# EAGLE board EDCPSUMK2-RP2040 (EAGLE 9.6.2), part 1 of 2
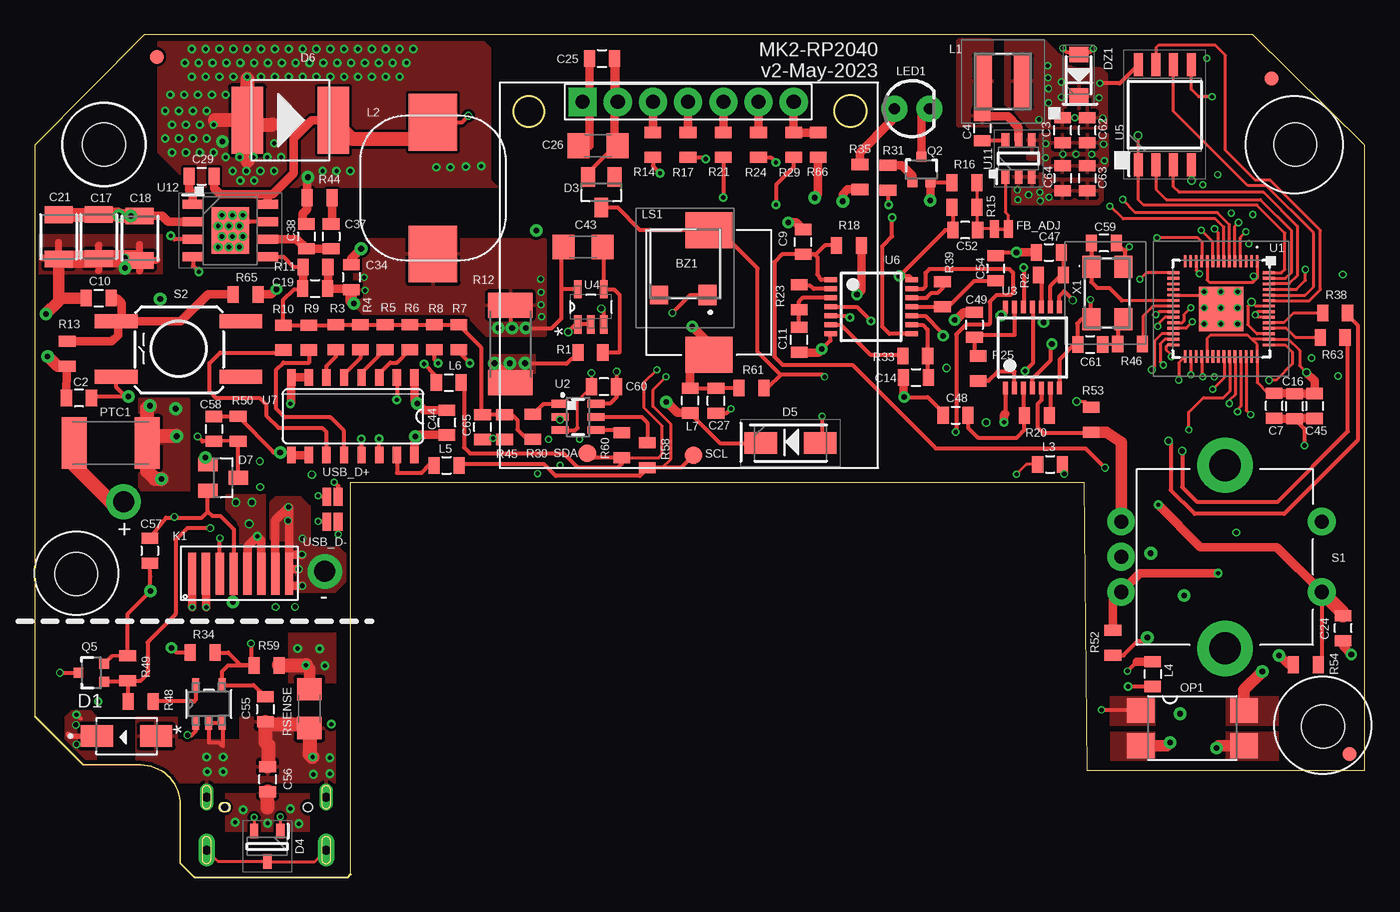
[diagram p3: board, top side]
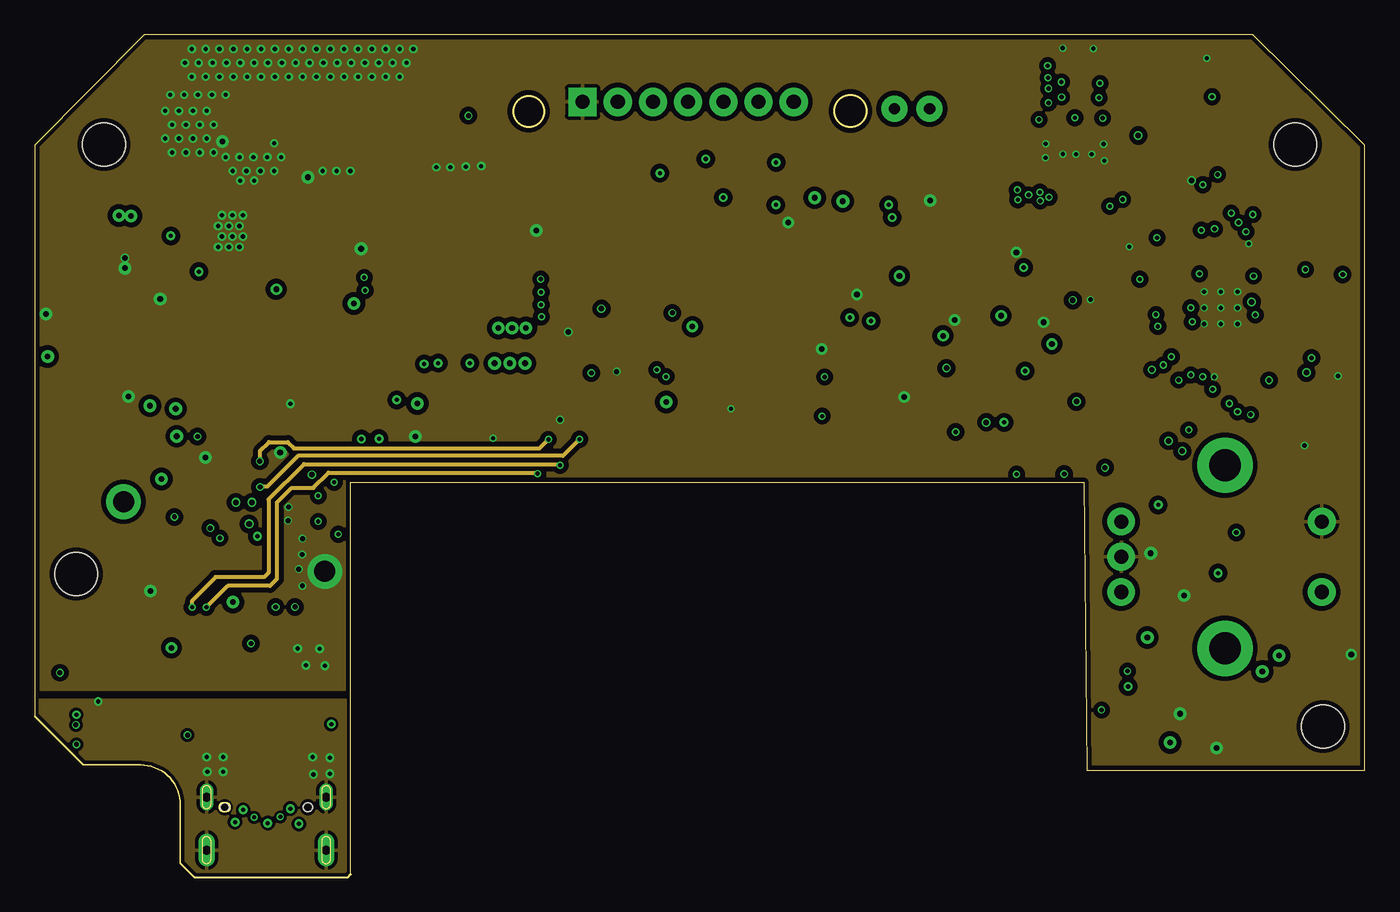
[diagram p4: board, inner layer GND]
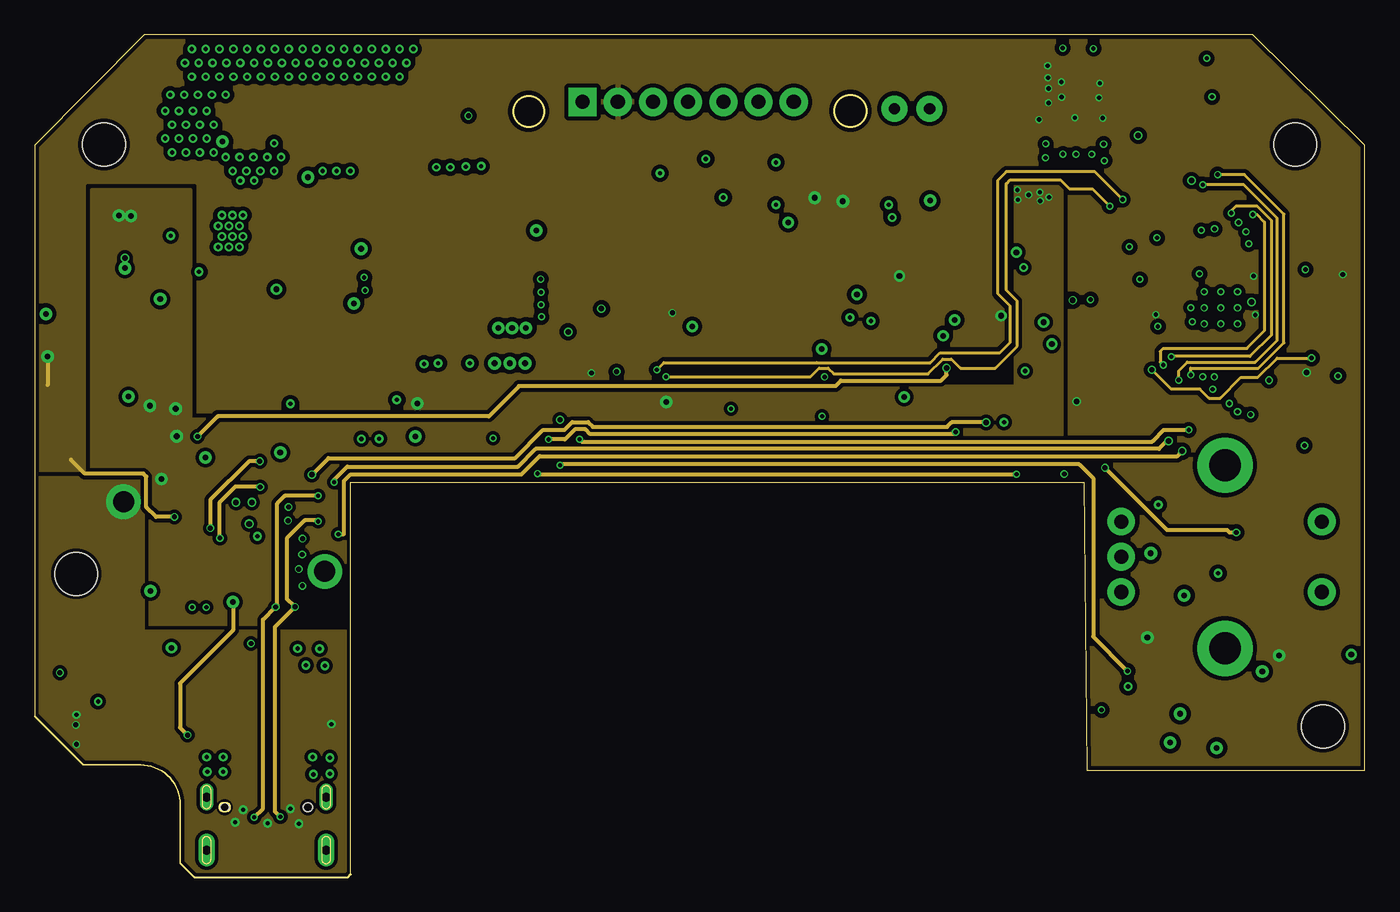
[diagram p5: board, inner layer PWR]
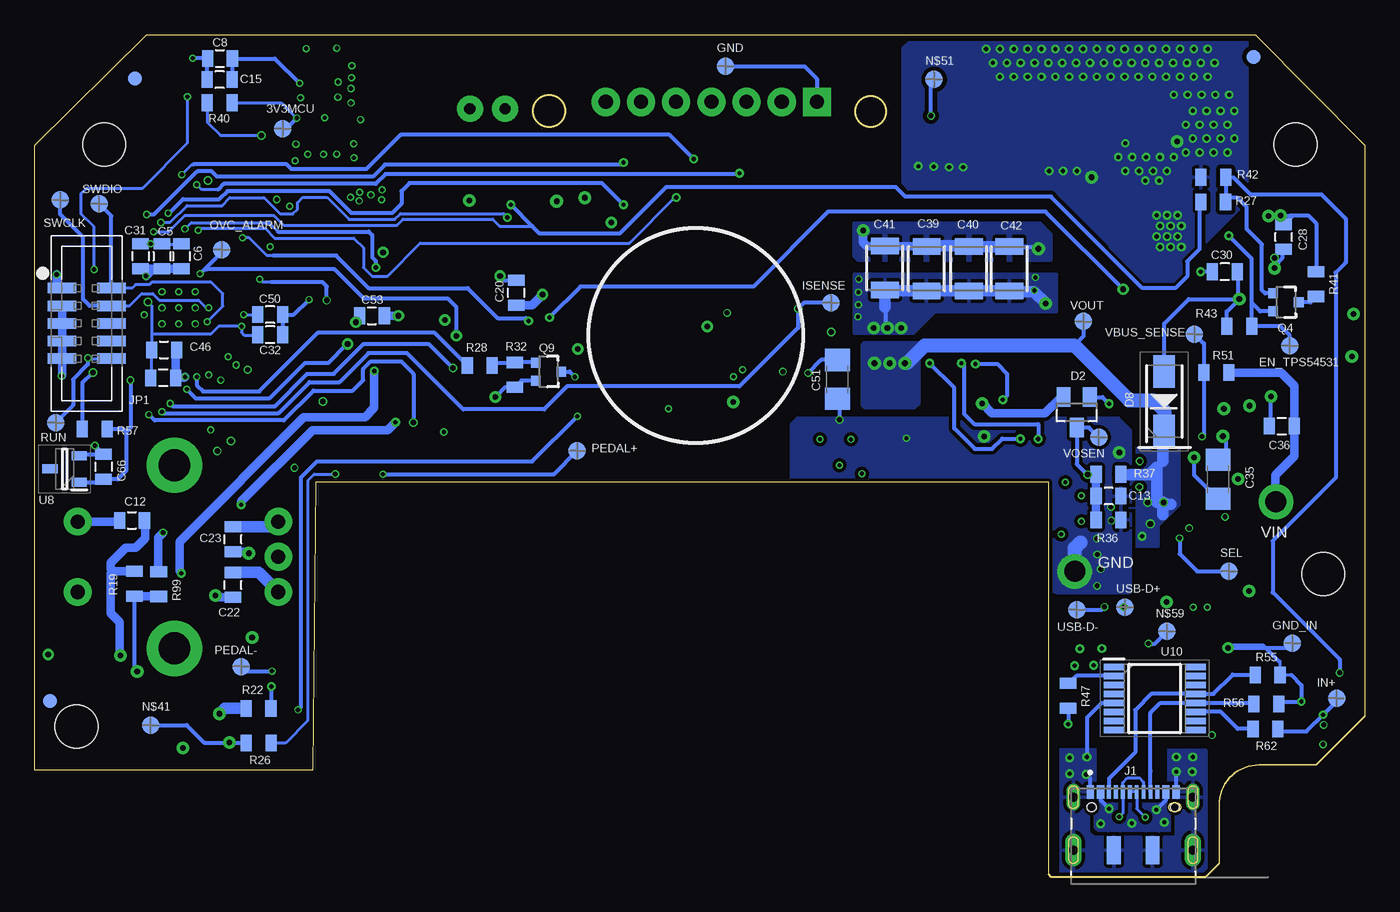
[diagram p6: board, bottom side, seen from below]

Size 96 x 60.8 mm. Coordinates in mm from the lower left corner, seen from the top.
Outline: 96,7.7 96,52.8 87.9,60.8 7.9,60.8 0,52.8 0,11.6 3.5,8.1 7.62,8.1 arc-90 10.5,5.22 10.5,1 11.5,0 22.6,0 22.8,0.2 22.8,28.5 75.71,28.5 75.92,7.7 96,7.7
Outline: circle at 35.64,55.26 radius 1.09
Outline: circle at 58.87,55.29 radius 1.14
Copper layers (1*2*15*16): Top 0.035mm / dielectric 0.2mm / GND 0.0175mm / dielectric 0.3mm / PWR 0.0175mm / dielectric 0.2mm / Bottom 0.035mm
Design rules "SeeedStudio_4layer_DRU_no_angle_20140221 *": minimum track width 8mil, minimum drill 12mil, track to track 8mil, track to pad 8mil, pad to pad 8mil, via to via 8mil, smd to smd 0mil, copper to edge 10mil, drill to drill 8mil, minimum pad ring 6mil, minimum via ring 4mil, stop-mask expansion 4mil, vias tented up to drill 25mil, thermal gap 10mil
Net classes: 1 vcc: width 0.254 mm
Holes 3.1 mm at 4.98,52.88 90.98,52.88 2.98,21.88 92.98,10.88
tRestrict: area 0.4,19.3 to 5.4,24.3; area 2.5,50.4 to 7.5,55.4; area 88.5,50.4 to 93.5,55.4; area 90.5,8.4 to 95.5,13.4
bRestrict: area 90.5,8.4 to 95.5,13.4; area 88.5,50.4 to 93.5,55.4; area 2.5,50.4 to 7.5,55.4; area 0.4,19.4 to 5.4,24.4

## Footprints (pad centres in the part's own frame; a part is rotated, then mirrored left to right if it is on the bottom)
TESTPAD_B1,27 = smd 1.27 x 1.27: TP 0,0
PKMCS0909 = smd 2.6 x 3.4: 1 -4.5,0; 2 4.5,0
0805 = smd 0.8 x 1.2: 1 -0.9,0; 2 0.9,0
1210 = smd 1.2 x 2: 1 -1.6,0; 2 1.6,0
1206 = smd 1.6 x 1.8: 1 -1.4,0; 2 1.4,0
DIOM4325X244N = smd 2.33 x 1.55: A 2.135,0; C -2.135,0
SOT23 = smd 1 x 1.4: 1 -0.95,-1.1; 2 0.95,-1.1; 3 0,1.1
SOT95P230X110-3N = smd 1.05 x 0.6: 1 -1.1,0.95; 2 -1.1,-0.95; 3 1.1,0
DIOM5226X244N = smd 2.35 x 1.55: 1 -2.15,0; 2 2.15,0
DO-214AB = smd 2.286 x 4.8: 1 -3.1,0; 2 3.1,0
SODFL3518X115N = smd 1.12 x 1.37: 1 -1.5,0; 2 1.5,0
SMT-JUMPER_2_NC_TRACE_NO-SILK = smd 0.635 x 1.27: 1 -0.508,0; 2 0.508,0
FIDUCIAL-1X2 = smd 1 x 1: 1 0,0
JAE_DX07S016JA1R1500 = smd 0.52 x 1: 1 -3.1,1.1; 2 -2.35,1.1; 11 2.35,1.1; 12 3.1,1.1 | smd 0.27 x 1: 3 -1.75,1.1; 4 -1.25,1.1; 5 -0.75,1.1; 6 -0.25,1.1; 7 0.25,1.1; 8 0.75,1.1; 9 1.25,1.1; 10 1.75,1.1 | smd 1 x 2: S1 -1.4,-3.1; S2 1.4,-3.1 | drill 0.65 long: S3 -4.32,0.725; S4 4.32,0.725 | drill 0.65 pad 1.2 long: S5 -4.32,-3.1; S6 4.32,-3.1 | hole 0.6: 3,0 | hole 0.63: 3,0; -3,0
OLED_LCD = drill 1.016 pad 2.032 square: 1 -7.42,13.7 | drill 1.016 pad 2.032: 2 -4.88,13.7; 3 -2.34,13.7; 4 0.2,13.7; 5 2.74,13.7; 6 5.28,13.7; 7 7.82,13.7
20021521-00010T1LF = smd 0.76 x 2.05: 1 -2.54,-1.78; 2 -2.54,1.78; 3 -1.27,-1.78; 4 -1.27,1.78; 5 0,-1.78; 6 0,1.78; 7 1.27,-1.78; 8 1.27,1.78; 9 2.54,-1.78; 10 2.54,1.78
FLEX8 = smd 0.6 x 3: 1 0.8,2.05; 2 1.8,2.05; 3 2.8,2.05; 4 3.8,2.05; 5 4.8,2.05; 7 5.8,2.05; 8 6.8,2.05; 9 7.8,2.05
NRS4018T100MDGJ = smd 1.2 x 3.7: 1 -1.4,0; 2 1.4,0
WE-LHMI = smd 4.1 x 3.5: 1 -4.75,0; 2 4.75,0
LED3MM = drill 0.813 pad 1.88: A -1.27,0; K 1.27,0
SMT0540SR = smd 1.5 x 1.3: 1 -2.25,-1.6; 2 2.25,-1.6 | smd 1.3 x 1.3: 3 -2.25,1.9
SMD4 = smd 1.78 x 2: 1 -1.27,-3.725; 2 1.27,-3.725; 3 1.27,3.725; 4 -1.27,3.725
1812L = smd 1.8 x 3.7: 1 -2.6,0; 2 2.65,0
SOT323 = smd 0.7 x 0.7: 1 -0.65,-0.925; 2 0.65,-0.925; 3 0,0.925
R2512 = smd 1.8 x 3.2: 1 -2.8,0; 2 2.8,0
ROTARY_ENC_PLAIN = drill 1.016 pad 2: A 7.493,-2.54; B 7.493,2.54; C 7.493,0; SW+ -6.985,2.54; SW- -6.985,-2.54 | drill 2.286 pad 4: P$3 0,6.604; P$4 0,-6.604
TAC_SW_SMD_KSC931G = smd 3.1 x 1: 1 -4.5,2; 2 4.5,2; 3 -4.5,-2; 4 4.5,-2
RP2040TR7 = smd 0.875 x 0.2: 1 -3.438,2.6; 2 -3.438,2.2; 3 -3.438,1.8; 4 -3.438,1.4; 5 -3.438,1; 6 -3.438,0.6; 7 -3.438,0.2; 8 -3.438,-0.2; 9 -3.438,-0.6; 10 -3.438,-1; 11 -3.438,-1.4; 12 -3.438,-1.8; 13 -3.438,-2.2; 14 -3.438,-2.6; 29 3.438,-2.6; 30 3.438,-2.2; 31 3.438,-1.8; 32 3.438,-1.4; 33 3.438,-1; 34 3.438,-0.6; 35 3.438,-0.2; 36 3.438,0.2; 37 3.438,0.6; 38 3.438,1; 39 3.438,1.4; 40 3.438,1.8; 41 3.438,2.2; 42 3.438,2.6 | smd 0.2 x 0.875: 15 -2.6,-3.438; 16 -2.2,-3.438; 17 -1.8,-3.438; 18 -1.4,-3.438; 19 -1,-3.438; 20 -0.6,-3.438; 21 -0.2,-3.438; 22 0.2,-3.438; 23 0.6,-3.438; 24 1,-3.438; 25 1.4,-3.438; 26 1.8,-3.438; 27 2.2,-3.438; 28 2.6,-3.438; 43 2.6,3.438; 44 2.2,3.438; 45 1.8,3.438; 46 1.4,3.438; 47 1,3.438; 48 0.6,3.438; 49 0.2,3.438; 50 -0.2,3.438; 51 -0.6,3.438; 52 -1,3.438; 53 -1.4,3.438; 54 -1.8,3.438; 55 -2.2,3.438; 56 -2.6,3.438 | smd 3.2 x 3.2: 57 0,0
SOT23-6 = smd 0.55 x 1.2: 1 0.95,1.3; 2 0,1.3; 3 -0.95,1.3; 4 -0.95,-1.3; 5 0,-1.3; 6 0.95,-1.3
TSSOP14 = smd 0.35 x 0.9: 1 -1.95,-2.925; 2 -1.3,-2.925; 3 -0.65,-2.925; 4 0,-2.925; 5 0.65,-2.925; 6 1.3,-2.925; 7 1.95,-2.925; 8 1.95,2.925; 9 1.3,2.925; 10 0.65,2.925; 11 0,2.925; 12 -0.65,2.925; 13 -1.3,2.925; 14 -1.95,2.925
SOT95P280X145-5N = smd 1.321 x 0.559: 1 -1.27,0.94; 2 -1.27,0; 3 -1.27,-0.94; 4 1.27,-0.94; 5 1.27,0.94
SOIC127P790X216-8N = smd 1.65 x 0.65: 1 -3.6,1.905; 2 -3.6,0.635; 3 -3.6,-0.635; 4 -3.6,-1.905; 5 3.6,-1.905; 6 3.6,-0.635; 7 3.6,0.635; 8 3.6,1.905
SO16 = smd 0.6 x 1.2: 1 -4.445,-2.8; 2 -3.175,-2.8; 3 -1.905,-2.8; 4 -0.635,-2.8; 5 0.635,-2.8; 6 1.905,-2.8; 7 3.175,-2.8; 8 4.445,-2.8; 9 4.445,2.8; 10 3.175,2.8; 11 1.905,2.8; 12 0.635,2.8; 13 -0.635,2.8; 14 -1.905,2.8; 15 -3.175,2.8; 16 -4.445,2.8
SOT96P240X120-3N = smd 1.1 x 0.65: 1 -1.05,0.96; 2 -1.05,-0.96; 3 1.05,0
21-0057F_MXM = smd 0.978 x 0.508: 1 -1.365,0.95; 2 -1.365,0; 3 -1.365,-0.95; 4 1.365,-0.95; 5 1.365,0.95
SOP65P640X120-16N = smd 1.475 x 0.45: 1 -2.938,2.275; 2 -2.938,1.625; 3 -2.938,0.975; 4 -2.938,0.325; 5 -2.938,-0.325; 6 -2.938,-0.975; 7 -2.938,-1.625; 8 -2.938,-2.275; 9 2.938,-2.275; 10 2.938,-1.625; 11 2.938,-0.975; 12 2.938,-0.325; 13 2.938,0.325; 14 2.938,0.975; 15 2.938,1.625; 16 2.938,2.275
SOT95P280X100-6N = smd 1.05 x 0.55: 1 -1.3,0.95; 2 -1.3,0; 3 -1.3,-0.95; 4 1.3,-0.95; 5 1.3,0; 6 1.3,0.95
SOIC127P600X163-9N = smd 1.5 x 0.65: 1 -2.7,1.905; 2 -2.7,0.635; 3 -2.7,-0.635; 4 -2.7,-1.905; 5 2.7,-1.905; 6 2.7,-0.635; 7 2.7,0.635; 8 2.7,1.905 | smd 2.71 x 3.35: 9 0,0
SMT-JUMPER_2_NO_NO-SILK = smd 0.635 x 1.27: 1 -0.406,0; 2 0.406,0
ABM3C16000MHZD4YT = smd 1.6 x 1.3: 1 -1.9,-1.15; 2 1.9,-1.15; 3 1.9,1.15; 4 -1.9,1.15

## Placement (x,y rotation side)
3V3MCU  TESTPAD_TPSQB1,27  [TESTPAD_B1,27]  78.11,54.02 0 bottom
BZ1  PKMCS0909E4000-R1  [PKMCS0909]  48.64,42.2 90 top
C2  100n 50v X7R/X5R  [0805]  3.18,34.58 180 top
C3  22uF 10V X5R  [0805]  74.18,53.9 90 top
C4  100n 50v X7R/X5R  [0805]  68.38,54.03 270 top
C5  100n 50v X7R/X5R  [0805]  86.81,44.8 270 bottom
C6  100n 50v X7R/X5R  [0805]  85.4,44.8 270 bottom
C7  100n 50v X7R/X5R  [0805]  89.45,34.01 90 top
C8  100n 50v X7R/X5R  [0805]  82.62,59.08 0 bottom
C9  1uF 50V X7R  [0805]  55.45,45.84 90 top
C10  100n 50v X7R/X5R  [0805]  4.61,41.78 0 top
C11  1uF 50V X7R  [0805]  55.16,38.79 90 top
C12  100n 50v X7R/X5R  [0805]  88.97,25.75 0 bottom
C13  1uF 50V X7R  [0805]  18.48,27.5 180 bottom
C14  100n 50v X7R/X5R  [0805]  63.6,36.06 0 top
C15  1uF 50V X7R  [0805]  82.65,57.55 180 bottom
C16  100n 50v X7R/X5R  [0805]  90.92,33.99 90 top
C17  4.7uF 50V X7R  [1210]  4.6,46.23 270 top
C18  4.7uF 50V X7R  [1210]  7.56,46.11 270 top
C19  N.C.  [0805]  20.22,42.47 0 top
C20  100n 50v X7R/X5R  [0805]  61.23,42.17 90 bottom
C21  4.7uF 50V X7R  [1210]  1.71,46.2 270 top
C22  100n 50v X7R/X5R  [0805]  81.69,21.09 90 bottom
C23  100n 50v X7R/X5R  [0805]  81.69,24.39 90 bottom
C24  100n 50v X7R/X5R  [0805]  94.44,17.98 90 top
C25  100n 50v X7R/X5R  [0805]  40.93,59.08 0 top
C26  10uF 50V X5R/X7R  [1206]  40.64,52.79 180 top
C27  100n 50v X7R/X5R  [0805]  49.16,34.38 90 top
C28  100n 50v X7R/X5R  [0805]  5.84,46.2 90 bottom
C29  100n 50v X7R/X5R  [0805]  12.03,50.58 0 top
C30  33n  [0805]  10.08,43.69 180 bottom
C31  100n 50v X7R/X5R  [0805]  88.35,44.8 270 bottom
C32  100n 50v X7R/X5R  [0805]  78.99,39.14 180 bottom
C33  100n 50v X7R/X5R  [0805]  86.73,36.03 180 bottom
C34  100n 50v X7R/X5R  [0805]  22.84,43.29 270 top
C35  10uF 50V X5R/X7R  [1206]  10.57,28.71 270 bottom
C36  100n 50v X7R/X5R  [0805]  5.98,32.55 0 bottom
C37  10nF  [0805]  21.38,46.23 270 top
C38  16pF  [0805]  19.59,46.23 270 top
C39  22uF 25V X5R  [1210]  31.61,43.91 90 bottom
C40  22uF 25V X5R  [1210]  28.56,43.91 90 bottom
C41  22uF 25V X5R  [1210]  34.62,43.96 90 bottom
C42  22uF 25V X5R  [1210]  25.64,43.91 90 bottom
C43  10uF 50V X5R/X7R  [1206]  39.56,45.47 0 top
C44  100n 50v X7R/X5R  [0805]  29.75,32.81 90 top
C45  1uF 50V X7R  [0805]  92.37,34 270 top
C46  1uF 50V X7R  [0805]  86.66,38.05 0 bottom
C47  100n 50v X7R/X5R  [0805]  73.2,45.09 0 top
C48  100n 50v X7R/X5R  [0805]  66.46,33.33 0 top
C49  100n 50v X7R/X5R  [0805]  67.82,39.86 270 top
C50  100n 50v X7R/X5R  [0805]  79.01,40.59 180 bottom
C51  10uF 50V X5R/X7R  [1206]  38.06,35.92 90 bottom
C52  N.C  [0805]  67.15,46.69 180 top
C53  100n 50v X7R/X5R  [0805]  71.65,40.52 0 bottom
C54  1uF 50V X7R  [0805]  69.35,43.93 270 top
C55  100n 50v X7R/X5R  [0805]  16.63,12.11 270 top
C56  1uF 50V X7R  [0805]  16.8,7.07 90 top
C57  100n 50v X7R/X5R  [0805]  8.29,23.55 270 top
C58  100n 50v X7R/X5R  [0805]  12.93,32.34 270 top
C59  27p  [0805]  77.16,45.76 180 top
C60  100n 50v X7R/X5R  [0805]  41.07,35.39 180 top
C61  27p  [0805]  76.17,38.44 0 top
C62  22uF 10V X5R  [0805]  75.96,53.9 90 top
C63  4.7uF 50V X5R  [0805]  75.96,50.43 270 top
C64  4.7uF 50V X5R  [0805]  74.18,50.44 270 top
C65  N.C.  [0805]  32.31,32.48 90 top
C66  100n 50v X7R/X5R  [0805]  91.02,29.61 270 bottom
D1  SMAJ24A  [DIOM4325X244N]  6.62,10.18 0 top
D2  BAV199  [SOT23]  20.77,33.54 180 bottom
D3  N.C  [SOT23]  40.88,49.43 180 top
D4  PESD5V0U2BT,215  [SOT95P230X110-3N]  16.77,2.22 270 top
D5  3SMAJ5923B-TP  [DIOM5226X244N]  54.54,31.32 0 top
D6  N.C  [DO-214AB]  18.43,54.62 0 top
D7  BAV199  [SOT23]  13.59,28.83 270 top
D8  RB060M-60TR  [DIOM5226X244N]  14.46,34.33 90 bottom
DZ1  MMSZ5228B-7-F  [SODFL3518X115N]  75.34,57.86 90 top
EN_TPS54531  TESTPAD_TPSQB1,27  [TESTPAD_B1,27]  5.41,38.35 0 bottom
FB_ADJ  JUMPER-SMT_2_NC_TRACE_NO-SILK  [SMT-JUMPER_2_NC_TRACE_NO-SILK]  69.77,46.77 0 top
FID1  FIDUCIAL1X2  [FIDUCIAL-1X2]  89.27,57.64 0 top
FID2  FIDUCIAL1X2  [FIDUCIAL-1X2]  94.9,8.89 0 top
FID3  FIDUCIAL1X2  [FIDUCIAL-1X2]  8.03,59.19 0 bottom
FID4  FIDUCIAL1X2  [FIDUCIAL-1X2]  8.79,59.19 0 top
FID5  FIDUCIAL1X2  [FIDUCIAL-1X2]  88.76,57.64 0 bottom
FID6  FIDUCIAL1X2  [FIDUCIAL-1X2]  94.9,12.7 0 bottom
GND  TESTPAD_TPSQB1,27  [TESTPAD_B1,27]  46.12,58.5 0 bottom
GND_IN  TESTPAD_TPSQB1,27  [TESTPAD_B1,27]  5.21,16.89 0 bottom
IN+  TESTPAD_TPSQB1,27  [TESTPAD_B1,27]  2.02,12.91 0 bottom
ISENSE  TESTPAD_TPSQB1,27  [TESTPAD_B1,27]  38.53,41.44 0 bottom
J1  DX07S016JA1R1500  [JAE_DX07S016JA1R1500]  16.7,5.05 0 bottom
J6  Display  [OLED_LCD]  46.95,42.24 0 top
JP1  20021521-00010T1LF  [20021521-00010T1LF]  92.24,39.96 270 bottom
K1  FLEX CONNECTORES  [FLEX8]  10.54,19.84 0 top
L1  NRS4018T4R7MDGJ  [NRS4018T100MDGJ]  69.87,57.42 0 top
L2  4.7uH  [WE-LHMI]  28.73,49.72 270 top
L3  MMZ2012Y202BT000  [0805]  73.28,29.79 0 top
L4  MMZ2012Y202BT000  [0805]  80.69,14.66 270 top
L5  MMZ2012Y202BT000  [0805]  29.7,29.71 0 top
L6  MMZ2012Y202BT000  [0805]  29.87,35.69 0 top
L7  MMZ2012Y202BT000  [0805]  47.3,34.4 90 top
LED1  [LED3MM]  63.31,55.45 0 top
LS1  SMT-0540-S-R  [SMT0540SR]  46.95,44.26 90 top
N$41  TESTPAD_TPSQB1,27  [TESTPAD_B1,27]  87.63,10.97 0 bottom
N$51  TESTPAD_TPSQB1,27  [TESTPAD_B1,27]  31.07,57.57 0 bottom
N$59  TESTPAD_TPSQB1,27  [TESTPAD_B1,27]  14.26,17.73 0 bottom
OP1  LTV816S  [SMD4]  83.54,10.76 270 top
OVC_ALARM  TESTPAD_TPSQB1,27  [TESTPAD_B1,27]  82.5,45.28 0 bottom
PEDAL+  TESTPAD_TPSQB1,27  [TESTPAD_B1,27]  56.83,30.76 0 bottom
PEDAL-  TESTPAD_TPSQB1,27  [TESTPAD_B1,27]  81.08,15.2 0 bottom
PTC1  2A NOM / 3.5A LIM  [1812L]  5.49,31.32 180 top
Q2  2N7002PW  [SOT323]  63.98,51.06 0 top
Q4  2N7002PW  [SOT323]  5.67,41.49 270 bottom
Q5  2N7002PW  [SOT323]  4.07,14.75 90 top
Q9  2N7002PW  [SOT323]  58.91,36.48 270 bottom
R1  10K  [0805]  40.09,37.86 180 top
R2  1K  [0805]  73.34,43.45 0 top
R3  11K  [0805]  21.72,38.95 90 top
R4  5K6  [0805]  23.49,38.95 90 top
R5  2K8  [0805]  25.27,38.95 90 top
R6  1K4  [0805]  27.05,38.95 90 top
R7  180K  [0805]  30.61,38.95 90 top
R8  91K  [0805]  28.83,38.95 90 top
R9  43K  [0805]  19.79,38.94 90 top
R10  22K  [0805]  17.93,38.94 90 top
R11  15K  [0805]  20.25,44.02 0 top
R12  0.025R / 1W  [R2512]  34.32,38.47 270 top
R13  2K2  [0805]  2.33,37.77 270 top
R14  33R  [0805]  44.6,52.84 90 top
R15  0R  [0805]  67.08,48.34 0 top
R16  N.C  [0805]  67.08,50.11 180 top
R17  33R  [0805]  47.14,52.84 90 top
R18  N.C  [0805]  58.75,45.58 180 top
R19  1K  [0805]  88.8,21.17 90 bottom
R20  1K  [0805]  72.33,33.32 180 top
R21  33R  [0805]  49.68,52.84 90 top
R22  330R  [0805]  79.84,12.17 180 bottom
R23  2K2  [0805]  55.16,41.84 270 top
R24  33R  [0805]  52.22,52.84 90 top
R25  1K  [0805]  68.1,36.71 90 top
R26  330R  [0805]  79.83,9.68 180 bottom
R27  1K  [0805]  10.93,48.72 180 bottom
R28  33R  [0805]  63.87,36.93 0 bottom
R29  33R  [0805]  54.76,52.84 90 top
R30  N.C  [0805]  35.95,32.51 270 top
R31  330R  [0805]  61.57,50.46 90 top
R32  10K  [0805]  61.34,36.24 270 bottom
R33  330R  [0805]  63.54,37.61 0 top
R34  N.C  [0805]  12.1,16.2 0 top
R35  130R  [0805]  59.55,50.52 90 top
R36  27K  [0805]  18.48,25.78 0 bottom
R37  150K  [0805]  18.48,29.07 180 bottom
R38  27R  [0805]  93.85,40.7 180 top
R39  10K  [0805]  65.51,42.05 270 top
R40  10K  [0805]  82.63,55.88 0 bottom
R41  150K  [0805]  3.49,42.8 90 bottom
R42  10K  [0805]  10.92,50.5 0 bottom
R43  11K  [0805]  9.04,39.76 0 bottom
R44  25K  [0805]  20.54,49.03 0 top
R45  N.C  [0805]  33.9,32.48 90 top
R46  1K  [0805]  79.05,38.47 180 top
R47  100R  [0805]  21.39,13.09 90 bottom
R48  100R  [0805]  7.63,12.68 180 top
R49  10K  [0805]  6.7,15.08 270 top
R50  56K  [0805]  14.66,32.36 90 top
R51  390K  [0805]  10.69,36.41 180 bottom
R52  2K2  [0805]  77.81,16.9 270 top
R53  2K2  [0805]  76.25,33.01 90 top
R54  2K2  [0805]  91.73,15.33 180 top
R55  5K1  [0805]  7,14.6 180 bottom
R56  5K1  [0805]  7.1,12.5 180 bottom
R57  330R  [0805]  91.65,32.35 180 bottom
R58  N.C  [0805]  44.21,30.45 90 top
R59  1K  [0805]  16.73,15.29 180 top
R60  N.C  [0805]  42.35,31.16 90 top
R61  330R  [0805]  51.73,35.3 180 top
R62  100K  [0805]  7.15,10.7 0 bottom
R63  27R  [0805]  93.67,38.94 180 top
R65  33R  [0805]  15.22,42.05 180 top
R66  10K  [0805]  56.53,52.84 90 top
R99  330R  [0805]  87.05,21.15 90 bottom
RSENSE  100mR  [1206]  19.81,12.16 90 top
RUN  TESTPAD_TPSQB1,27  [TESTPAD_B1,27]  94.48,32.8 0 bottom
S1  ROTARTY_ENCODER  [ROTARY_ENC_PLAIN]  85.9,23.12 180 top
S2  [TAC_SW_SMD_KSC931G]  10.37,38.1 180 top
SCL  TESTPAD_TPSQB1,27  [TESTPAD_B1,27]  47.55,30.46 0 top
SDA  TESTPAD_TPSQB1,27  [TESTPAD_B1,27]  39.87,30.58 0 top
SEL  TESTPAD_TPSQB1,27  [TESTPAD_B1,27]  9.8,22.06 0 bottom
SWCLK  TESTPAD_TPSQB1,27  [TESTPAD_B1,27]  94.14,48.89 0 bottom
SWDIO  TESTPAD_TPSQB1,27  [TESTPAD_B1,27]  91.35,48.6 0 bottom
U1  RP2040TR7  [RP2040TR7]  85.62,41.01 270 top
U2  MCP4725  [SOT23-6]  39.2,33.21 90 top
U3  SN74AC14PWR  [TSSOP14]  72.01,38.22 0 top
U4  MAX9938FEUK+T  [SOT95P280X145-5N]  40.13,41.15 90 top
U5  W25Q64JVSSIQ  [SOIC127P790X216-8N]  81.55,55.02 90 top
U6  SN74AC14PWR  [TSSOP14]  60.35,41.15 270 top
U7  TPIC2810D  [SO16]  22.95,33.26 180 top
U8  LM4040C30FTA  [SOT96P240X120-3N]  93.84,29.46 180 bottom
U9  MAX9064EUK+T  [21-0057F_MXM]  12.55,12.5 90 top
U10  IP2721  [SOP65P640X120-16N]  15.15,12.9 0 bottom
U11  AP63203  [SOT95P280X100-6N]  71,51.86 90 top
U12  AP64501SP-13  [SOIC127P600X163-9N]  14.1,46.66 0 top
USB-D+  TESTPAD_TPSQB1,27  [TESTPAD_B1,27]  17.31,19.48 0 bottom
USB-D-  TESTPAD_TPSQB1,27  [TESTPAD_B1,27]  20.78,19.31 0 bottom
USB_D+  JUMPER-SMT_2_NO_NO-SILK  [SMT-JUMPER_2_NO_NO-SILK]  21.47,27.45 180 top
USB_D-  JUMPER-SMT_2_NO_NO-SILK  [SMT-JUMPER_2_NO_NO-SILK]  21.47,25.65 180 top
VBUS_SENSE  TESTPAD_TPSQB1,27  [TESTPAD_B1,27]  12.27,39.19 0 bottom
VOSEN  TESTPAD_TPSQB1,27  [TESTPAD_B1,27]  19.19,31.75 0 bottom
VOUT  TESTPAD_TPSQB1,27  [TESTPAD_B1,27]  20.29,40.1 0 bottom
X1  ABM3C-12.000MHZ-D4Y-T  [ABM3C16000MHZD4YT]  77.4,42.16 270 top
